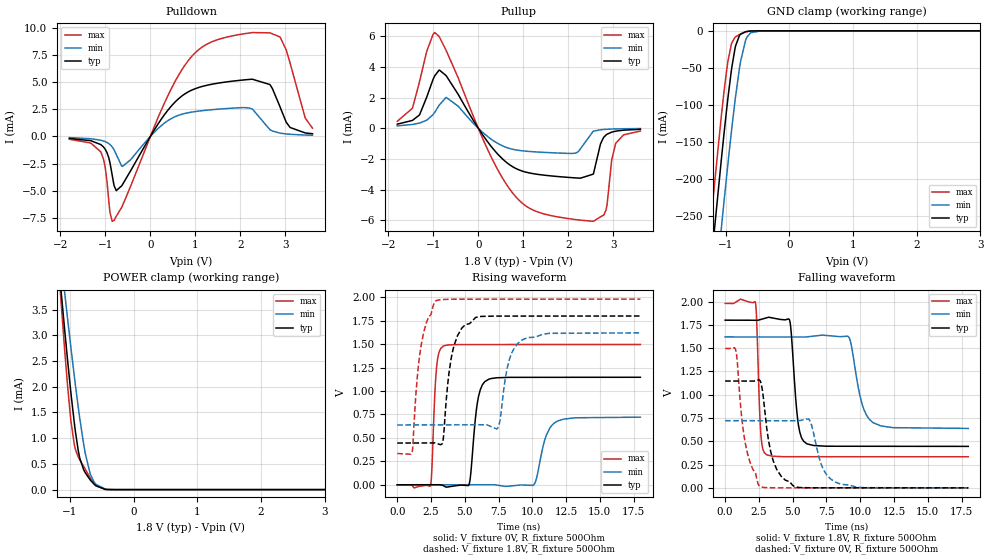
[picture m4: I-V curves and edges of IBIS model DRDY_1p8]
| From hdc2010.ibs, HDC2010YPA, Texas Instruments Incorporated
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[Model]   DRDY_1p8
Model_type   I/O
Polarity   Non-Inverting
Enable   Active-Low
Vinl = .54
Vinh = 1.26
Vmeas = 0.9
Vref = 1.8
Cref = 15pF
Rref = 500
|   typ   min   max
|   (nom PVT)   (slow PVT)   (fast PVT)
C_comp   0.887p   0.876p   0.898p
|C_comp (ON state)   0.913p   0.891p   0.940p
|C_comp (OFF state)   0.887p   0.876p   0.898p
[Model spec]
|subparameter
Vinl   0.54   0.486   0.594
Vinh   1.26   1.134   1.386
[Voltage Range]   1.8   1.62   1.98
[Temperature Range]   27   125   -40
[Pullup Reference]   1.8   1.62   1.98
[Pulldown Reference]   0   -0   -0
[Power Clamp Reference]   1.8   1.62   1.98
[GND Clamp Reference]   0   0   0
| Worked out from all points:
|   slope of the pulldown table from 0 to 0.27 V, typ, clamps not added: 154 ohm
|   slope of the pullup table from 0 to 0.27 V, typ, clamps not added: 240 ohm
|   GND clamp passes 1 mA (typ) near -0.68 V on its own axis
|   POWER clamp passes 1 mA (typ) near -0.90 V on its own axis
|   falling waveform, V_fixture 1.8V, R_fixture 500Ohm: 20-80 % time 426ps typ, 823ps min, 238ps max; typ from 1.8 V to 0.445 V
|   rising waveform, V_fixture 0V, R_fixture 500Ohm: 20-80 % time 475ps typ, 774ps min, 280ps max; typ from 0 V to 1.15 V
|   rising waveform, V_fixture 1.8V, R_fixture 500Ohm: 20-80 % time 782ps typ, 799ps min, 758ps max; typ from 0.445 V to 1.8 V
|   falling waveform, V_fixture 0V, R_fixture 500Ohm: 20-80 % time 862ps typ, 937ps min, 815ps max; typ from 1.15 V to 0 V
[Pulldown]
|   Voltage   I(typ)   I(min)   I(max)
-1.8V     -188.9uA   -112.8uA   -263.1uA
-1.103V   -751.4uA   -354.9uA   -1.417mA
-1.001V   -1.208mA   -490.2uA   -2.936mA
-898.2mV  -2.421mA   -749.7uA   -7.002mA
-806.4mV  -4.546mA   -1.237mA   -7.73mA
-622.8mV  -4.46mA    -2.768mA   -6.407mA
840.6mV   4.101mA    2.178mA    6.978mA
2.266V    5.264mA    2.514mA    9.56mA
2.655V    4.77mA     615.3uA    9.532mA
2.882V    2.684mA    296.4uA    9.138mA
3.103V    819.3uA    191.7uA    6.738mA
3.6V      244.1uA    105.4uA    757.5uA
[GND Clamp]
|   Voltage   I(typ)   I(min)   I(max)
-1.8V     -855.6mA   -946.4mA   -797.6mA
-1.228V   -314.1mA   -408.2mA   -253.4mA
-1.179V   -270.2mA   -364.2mA   -209.6mA
-1.071V   -175.6mA   -268.6mA   -116.8mA
-1.028V   -139.6mA   -231.5mA   -82.96mA
-963mV    -89.09mA   -177.6mA   -39.96mA
-914.4mV  -55.65mA   -139.1mA   -19.12mA
-855mV    -24.2mA    -95.28mA   -8.854mA
-784.8mV  -6.422mA   -51.06mA   -5.084mA
-666mV    -812.8uA   -8.529mA   -988uA
-444.6mV  -3.031uA   -66.8uA    -699.2nA
3.6V      0A         0A         0A
[Pullup]
|   Voltage   I(typ)   I(min)   I(max)
-1.8V     267.7uA    155.9uA    451.7uA
-1.465V   508.2uA    246.3uA    1.3mA
-968.4mV  3.414mA    1.035mA    6.24mA
-714.6mV  3.433mA    2.013mA    5.078mA
235.8mV   -994.8uA   -601.5uA   -1.563mA
813.6mV   -2.593mA   -1.401mA   -4.404mA
2.153V    -3.236mA   -1.621mA   -5.952mA
2.552V    -2.993mA   -195.8uA   -6.067mA
2.839V    -435.2uA   -68.62uA   -5.313mA
2.963V    -252.9uA   -51.39uA   -2.073mA
3.055V    -188.4uA   -42.96uA   -969.7uA
3.6V      -68.17uA   -20.57uA   -180.6uA
[POWER Clamp]
|   Voltage   I(typ)   I(min)   I(max)
-1.8V     13.39mA    12.36mA    15.82mA
-1.184V   4.472mA    4.985mA    4.409mA
-1.087V   3.162mA    3.88mA     2.78mA
-1.039V   2.536mA    3.342mA    2.04mA
-995.4mV  2.006mA    2.874mA    1.465mA
-925.2mV  1.235mA    2.143mA    841.7uA
-844.2mV  606.8uA    1.37mA     575.1uA
-757.8mV  325.8uA    694.2uA    394.5uA
-682.2mV  189.3uA    309.5uA    230.3uA
-590.4mV  73.01uA    101uA      81.2uA
-336.6mV  220.5nA    1.211uA    52.78nA
3.6V      0A         0A         0A
[Ramp]
R_load = 500
|   typ   min   max
dV/dt_r   0.68794/4.74704e-10   0.432623/7.5795e-10   0.897585/2.78681e-10
dV/dt_f   0.812854/4.2328e-10   0.589185/8.2175e-10   0.987799/2.35223e-10
[Falling Waveform]
V_fixture = 1.8V
V_fixture_min = 1.62V
V_fixture_max = 1.98V
R_fixture = 500Ohm
C_fixture = 0F
|   Time   V(typ)   V(min)   V(max)
0s        1.8V       1.62V      1.98V
2.237ns   1.799V     1.62V      1.994V
2.634ns   1.807V     1.62V      594.7mV
3.051ns   1.825V     1.62V      357.2mV
4.764ns   1.804V     1.619V     334.3mV
5.401ns   698.3mV    1.619V     334.3mV
6.025ns   475.5mV    1.62V      334.2mV
9.183ns   446.6mV    1.612V     334.1mV
10.96ns   446.3mV    699.7mV    334mV
18ns      445.2mV    638mV      333.7mV
[Rising Waveform]
V_fixture = 0V
V_fixture_min = 0V
V_fixture_max = 0V
R_fixture = 500Ohm
C_fixture = 0F
|   Time   V(typ)   V(min)   V(max)
0s        980.8pV    39.49nV    -104.6pV
2.458ns   345.5uV    142uV      -11.02mV
2.896ns   407.1uV    167.2uV    1.225V
3.404ns   -8.301mV   196.6uV    1.478V
5.301ns   -3.096mV   306.1uV    1.495V
5.973ns   908.7mV    344.9uV    1.495V
6.761ns   1.125V     390.4uV    1.495V
10.07ns   1.146V     -4.061mV   1.496V
11.88ns   1.146V     679.9mV    1.496V
18ns      1.147V     721mV      1.496V
[Rising Waveform]
V_fixture = 1.8V
V_fixture_min = 1.62V
V_fixture_max = 1.98V
R_fixture = 500Ohm
C_fixture = 0F
|   Time   V(typ)   V(min)   V(max)
0s        445.1mV    637.9mV    333.6mV
1.097ns   445.5mV    638.2mV    343.1mV
1.755ns   445.7mV    638.4mV    1.475V
2.878ns   443mV      638.8mV    1.964V
3.376ns   463.2mV    639mV      1.976V
4.199ns   1.482V     639.2mV    1.979V
5.793ns   1.783V     639.7mV    1.979V
7.436ns   1.799V     603.2mV    1.979V
9.238ns   1.799V     1.544V     1.979V
18ns      1.8V       1.62V      1.98V
[Falling Waveform]
|Gnd
V_fixture = 0V
V_fixture_min = 0V
V_fixture_max = 0V
R_fixture = 500Ohm
C_fixture = 0F
|   Time   V(typ)   V(min)   V(max)
0s        1.147V     721.2mV    1.496V
783.1ps   1.147V     721.1mV    1.478V
1.481ns   1.146V     721mV      488.5mV
2.597ns   1.148V     720.8mV    12.52mV
3.554ns   292.9mV    720.6mV    1.233mV
5.14ns    13.07mV    720.3mV    474.1uV
6.235ns   1.081mV    729.9mV    439.5uV
7.275ns   711uV      196.6mV    406.7uV
8.572ns   634.6uV    38.58mV    365.7uV
18ns      79.35uV    45.91uV    68.1uV
